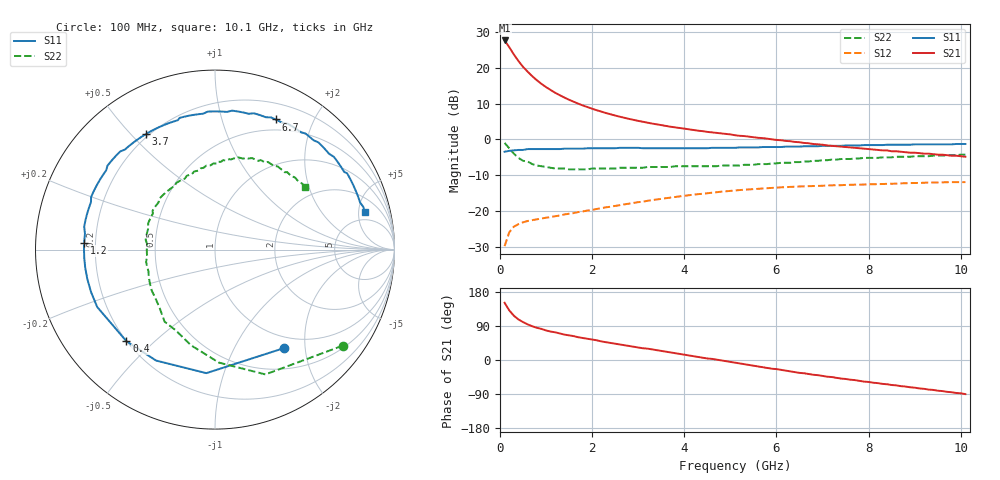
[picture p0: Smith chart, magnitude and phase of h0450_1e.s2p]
!HBFP-0450
!S and NOISE PARAMETERS at Vce=1V  Ic=15mA.  LAST UPDATED  09-04-98
# GHZ S MA R  50
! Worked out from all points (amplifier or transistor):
!   101 points, 100 MHz to 10.1 GHz, reference 50 ohm
!   highest |S21| = 27.7 dB at 100 MHz (marker M1)
!   |S21| within 3 dB of that: start of sweep to 255.6 MHz
!   unconditionally stable (mu >= 1): 2.431 GHz to 2.595 GHz; 2.605 GHz to end of sweep
!   at 1.7 GHz: K = 0.85, MSG = 15.2 dB, |S12| = -20.4 dB
!   at 5.1 GHz: K = 1.15, MAG = 5.4 dB, |S12| = -14.3 dB
!   at 10.1 GHz: K = 1.10, MAG = 1.7 dB, |S12| = -12.0 dB
!   lowest NFmin = 1.20 dB at 1.8 GHz
!   S11 on the Smith chart (normalised r, x): 100 MHz: 0.81, -1.61; 400 MHz: 0.20, -0.41; 1.2 GHz: 0.16, +0.03; 3.7 GHz: 0.19, +0.55; 6.7 GHz: 0.37, +1.50; 10.1 GHz: 3.68, +5.89
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0.1  0.67 -55.0  24.14 151.0  0.032 66.0  0.89 -37.0
0.2  0.69 -94.0  19.47 131.0  0.05 49.0  0.75 -68.0
0.3  0.7 -118.0  15.4 117.0  0.06 39.0  0.63 -88.0
0.4  0.71 -134.0  12.45 107.0  0.065 34.0  0.55 -104.0
0.5  0.71 -145.0  10.32 100.0  0.069 30.0  0.5 -116.0
0.6  0.73 -154.0  8.83 94.0  0.072 27.0  0.49 -125.0
0.7  0.73 -161.0  7.63 89.0  0.074 26.0  0.45 -133.0
0.8  0.73 -167.0  6.7 85.0  0.076 26.0  0.43 -140.0
0.9  0.73 -172.0  5.96 82.0  0.078 25.0  0.42 -147.0
1  0.73 -176.0  5.37 78.0  0.08 25.0  0.41 -152.0
1.2  0.73 177.0  4.47 73.0  0.084 25.0  0.39 -162.0
1.4  0.74 170.0  3.83 67.0  0.089 25.0  0.39 -170.0
1.8  0.74 159.0  2.97 58.0  0.098 25.0  0.38 177.0
2.2  0.75 150.0  2.44 49.0  0.109 24.0  0.39 167.0
2.5  0.75 144.0  2.15 43.0  0.117 22.0  0.39 161.0
3.5  0.75 125.0  1.58 24.0  0.147 15.0  0.41 143.0
3.7  0.75 121.0  1.5 20.0  0.153 13.0  0.41 140.0
5.1  0.76 95.0  1.14 -7.0  0.192 -3.0  0.43 115.0
6.7  0.8 65.0  0.88 -37.0  0.221 -25.0  0.49 86.0
6.8  0.8 64.0  0.86 -39.0  0.222 -27.0  0.5 85.0
8.5  0.84 37.0  0.68 -66.0  0.239 -49.0  0.56 60.0
10.1  0.86 14.0  0.57 -90.0  0.252 -71.0  0.61 35.0
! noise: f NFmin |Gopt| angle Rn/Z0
1.8  1.2  0.52  -170  0.04
2  1.25  0.53  -166  0.05
2.5  1.36  0.56  -155  0.07
3.5  1.66  0.62  -133  0.18
4  1.83  0.65  -121  0.28
5  2.08  0.69  -100  0.6
5.5  2.28  0.71  -90  0.84
7  2.65  0.76  -61  1.86
8  3.03  0.78  -44  2.71
10  3.49  0.81  -14  4.34
